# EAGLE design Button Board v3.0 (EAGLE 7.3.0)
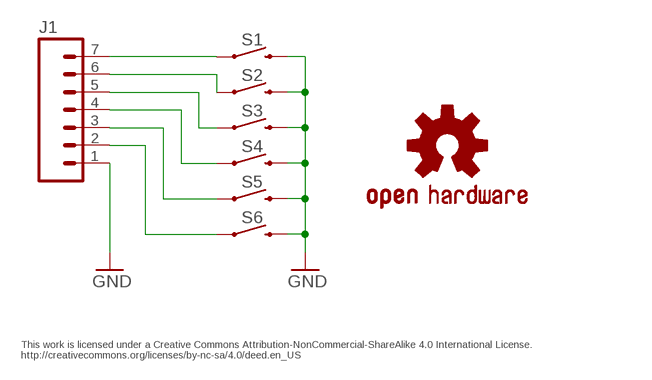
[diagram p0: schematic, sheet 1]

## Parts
J1  M07  [1X07]
S1  MOMENTARY-SWITCH-SPST-PTH-12MM  [TACTILE_SWITCH_PTH_12MM]
S2  MOMENTARY-SWITCH-SPST-PTH-12MM  [TACTILE_SWITCH_PTH_12MM]
S3  MOMENTARY-SWITCH-SPST-PTH-12MM  [TACTILE_SWITCH_PTH_12MM]
S4  MOMENTARY-SWITCH-SPST-PTH-12MM  [TACTILE_SWITCH_PTH_12MM]
S5  MOMENTARY-SWITCH-SPST-PTH-12MM  [TACTILE_SWITCH_PTH_12MM]
S6  MOMENTARY-SWITCH-SPST-PTH-12MM  [TACTILE_SWITCH_PTH_12MM]
U$7  OSHW-LOGOS  [OSHW-LOGO-S]

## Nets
GND: J1.1 S1.3 S2.3 S3.3 S4.3 S5.3 S6.3
N$1: J1.7 S1.1
N$3: J1.6 S2.1
N$5: J1.5 S3.1
N$7: J1.4 S4.1
N$9: J1.3 S5.1
N$18: J1.2 S6.1

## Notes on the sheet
- This work is licensed under a Creative Commons Attribution-NonCommercial-ShareAlike 4.0 International License.
  http://creativecommons.org/licenses/by-nc-sa/4.0/deed.en_US

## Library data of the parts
J1 = SparkFun-Connectors:M07: Header 7 Standard 7-pin 0.1" header. Use with straight break away headers (SKU : PRT-00116), right angle break away headers (PRT-00553), swiss pins (PRT-00743), machine pins (PRT-00117), and female headers (PRT-00115). NOTES ON THE VARIANTS LOCK and LOCK_LONGPADS... This footprint was designed to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
S1-S6 = SparkFun-Switches:MOMENTARY-SWITCH-SPST: Momentary Switch (Pushbutton) - SPST; PROD_ID: SWCH-09185; SF_SKU: COM-09190
U$7 = SparkFun:OSHW-LOGO: Open Source Hardware Logo This logo indicates the piece of hardware it is found on incorporates a OSHW license and/or adheres to the definition of open source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

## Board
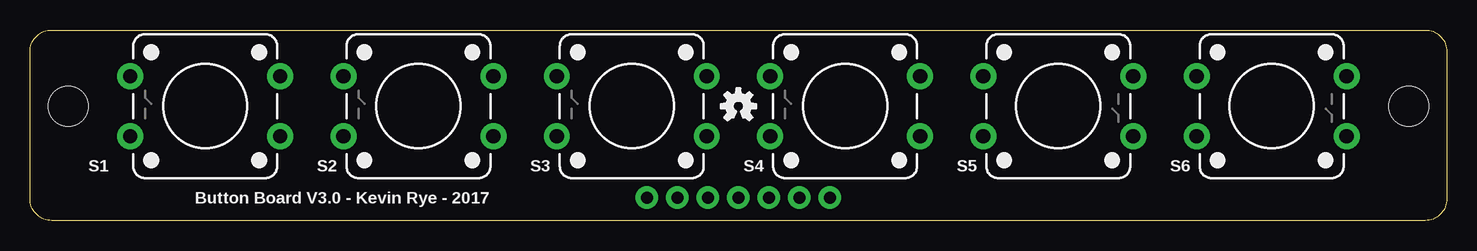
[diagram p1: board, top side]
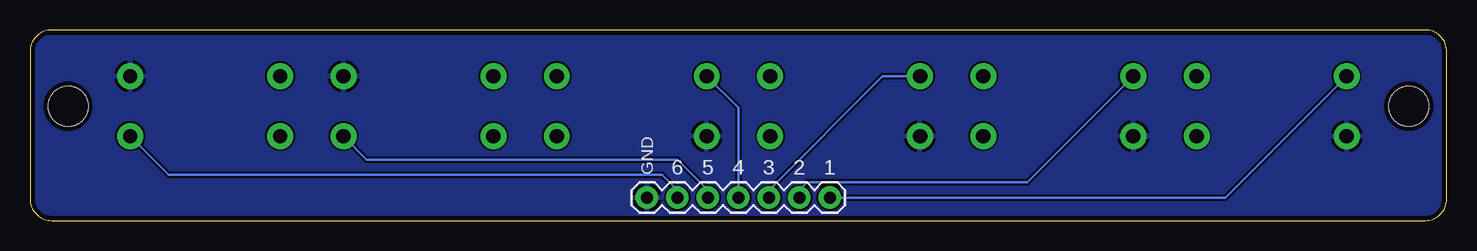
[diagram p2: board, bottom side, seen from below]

Size 118.11 x 15.88 mm. Coordinates in mm from the lower left corner, seen from the top.
Outline: 1.8,15.88 116.31,15.88 arc-90 118.11,14.08 118.11,1.8 arc-90 116.31,0 1.8,0 arc-90 0,1.8 0,14.08 arc-90 1.8,15.88
Copper layers (1*16): Top 0.0356mm / dielectric 1.5011mm / Bottom 0.0356mm
Design rules "LaenPCBOrder": minimum track width 6mil, minimum drill 13mil, track to track 6mil, track to pad 6mil, pad to pad 6mil, via to via 6mil, smd to smd 6mil, copper to edge 15mil, drill to drill 6mil, minimum pad ring 7mil, minimum via ring 7mil, stop-mask expansion 3mil, vias tented up to drill 0mil, thermal gap 10mil

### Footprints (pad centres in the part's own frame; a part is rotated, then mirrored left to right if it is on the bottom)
1X07 = drill 1.016 pad 1.88: 1 0,0; 2 2.54,0; 3 5.08,0; 4 7.62,0; 5 10.16,0; 6 12.7,0; 7 15.24,0
TACTILE_SWITCH_PTH_12MM = drill 1.2 pad 2.159: 1 6.25,-2.5; 2 -6.25,-2.5; 3 6.25,2.5; 4 -6.25,2.5
STAND-OFF = hole 3.302: 0,0

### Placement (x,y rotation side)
J1  66.67,1.91 0 bottom
S1  14.6,9.53 180 top
S2  32.38,9.53 180 top
S3  50.16,9.53 180 top
S4  67.95,9.53 180 top
S5  85.72,9.53 0 top
S6  103.5,9.53 0 top
U$1  [STAND-OFF]  3.17,9.53 0 top
U$2  [STAND-OFF]  114.94,9.53 0 top
U$7  59.05,9.53 0 top

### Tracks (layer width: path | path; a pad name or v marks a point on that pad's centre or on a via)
GND
  pour Bottom: 0,16.51 118.11,16.51 118.11,-0.64 0,-0.64
N$1
  Bottom 0.229: S1.1 18.48,1.91 J1.7
N$3
  Bottom 0.229: S2.1 34.98,3.17 53.34,3.17 53.98,2.54 J1.6
N$5
  Bottom 0.229: S3.1 47.03,12.03 56.52,2.54 J1.5
N$7
  Bottom 0.229: S4.1 59.05,9.38 J1.4
N$9
  Bottom 0.229: S5.1 90.03,5.08 64.13,5.08 61.59,2.54 J1.3
N$18
  Bottom 0.229: S6.1 106.54,3.81 65.41,3.81 64.13,2.54 J1.2

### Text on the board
Unrouted: This work is licensed under a Creative Commons Attribution-NonCommercial-ShareAlike 4.0 International License. / http://creativecommons.org/licenses/by-nc-sa/4.0/deed.en_US
tNames: Button Board V3.0 - Kevin Rye - 2017
bNames: 1 | 2 | 3 | 4 | 5 | 6 | GND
